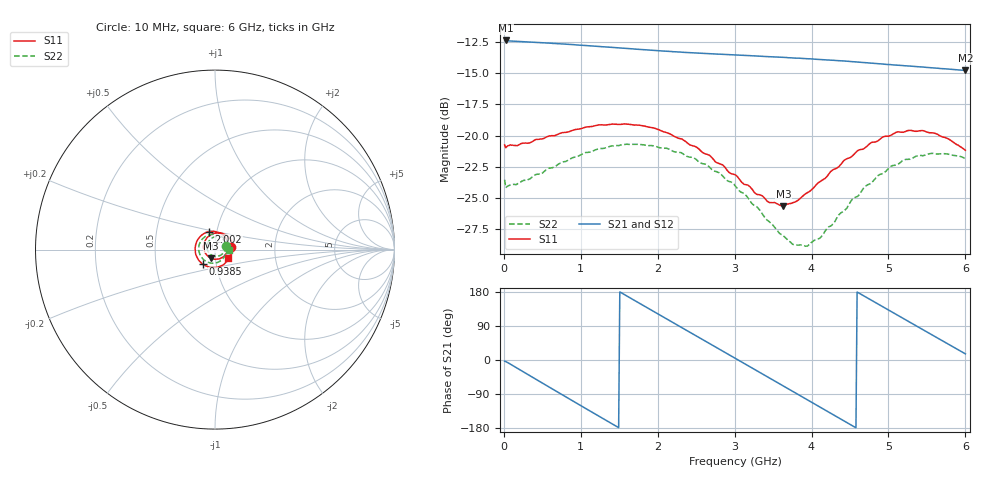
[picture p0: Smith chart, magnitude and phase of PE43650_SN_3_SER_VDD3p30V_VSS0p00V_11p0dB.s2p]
!Keysight Technologies,N5245B,MY57181451,A.13.50.07
!Date: Tuesday, May 07, 2019 08:00:07
!Correction: S11(Full 2 Port(1,2))
!S21(Full 2 Port(1,2))
!S12(Full 2 Port(1,2))
!S22(Full 2 Port(1,2))
!S2P File: Measurements: S11, S21, S12, S22:
# Hz S  dB  R 50
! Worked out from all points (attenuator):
!   401 points, 10 MHz to 6 GHz, reference 50 ohm
!   highest |S21| = -12.38 dB at 24.98 MHz (marker M1); lowest = -14.8 dB at 6 GHz (marker M2)
!   lowest |S11| = -25.6 dB at 3.634 GHz (marker M3), VSWR 1.11, Z = 47.7 - j4.58 ohm
!   |S11| at or under -10 dB: start of sweep to end of sweep
!   |S22| runs from -28.9 to -20.7 dB; largest |S21 - S12| = 0.0017
!   S11 on the Smith chart (normalised r, x): 10 MHz: 1.20, +0.04; 938.5 MHz: 0.86, -0.14; 2.002 GHz: 0.92, +0.19; 6 GHz: 1.16, -0.10
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1e7  -20.75 9.7  -12.38 -3.2  -12.44 -3.3  -23.55 16.8
2.4975e7  -20.98 1.3  -12.38 -4.2  -12.44 -4.1  -24.18 4.3
2.64575e8  -20.61 -39.0  -12.48 -32.5  -12.54 -32.5  -23.58 -38.2
5.1915e8  -20.24 -75.2  -12.58 -63.1  -12.62 -63.1  -22.91 -74.5
9.3845e8  -19.51 -129.7  -12.74 -113.1  -12.79 -113.1  -21.70 -126.2
1.013325e9  -19.43 -139.0  -12.77 -121.9  -12.82 -122.0  -21.50 -135.2
1.2679e9  -19.14 -168.9  -12.88 -152.1  -12.93 -152.1  -21.04 -162.9
1.492525e9  -19.11 165.1  -12.97 -178.5  -13.03 -178.5  -20.81 173.4
1.732125e9  -19.17 138.4  -13.09 153.3  -13.14 153.3  -20.71 149.0
2.001675e9  -19.51 109.0  -13.20 121.8  -13.25 121.8  -20.93 122.5
2.01665e9  -19.54 107.4  -13.21 120.0  -13.26 120.1  -20.95 120.9
2.4659e9  -20.84 56.4  -13.38 67.7  -13.43 67.7  -21.79 76.0
2.750425e9  -22.11 23.0  -13.47 34.5  -13.52 34.5  -22.88 46.3
3.005e9  -23.14 -11.2  -13.54 4.8  -13.60 4.9  -24.02 18.5
3.289525e9  -24.72 -53.7  -13.63 -28.4  -13.68 -28.3  -25.72 -18.0
3.63395e9  -25.64 -113.7  -13.74 -68.6  -13.78 -68.6  -28.05 -70.6
3.7837e9  -25.34 -140.3  -13.79 -86.1  -13.84 -86.1  -28.73 -98.0
4.008325e9  -24.30 -177.4  -13.86 -112.4  -13.92 -112.4  -28.53 -141.0
4.517475e9  -21.71 113.7  -14.08 -171.9  -14.12 -171.8  -25.20 138.9
5.01165e9  -20.03 59.7  -14.31 130.6  -14.36 130.8  -22.58 83.6
5.475875e9  -19.66 14.8  -14.53 76.8  -14.58 76.9  -21.58 40.2
6e9  -21.18 -31.1  -14.78 16.2  -14.83 16.3  -21.86 -2.4
